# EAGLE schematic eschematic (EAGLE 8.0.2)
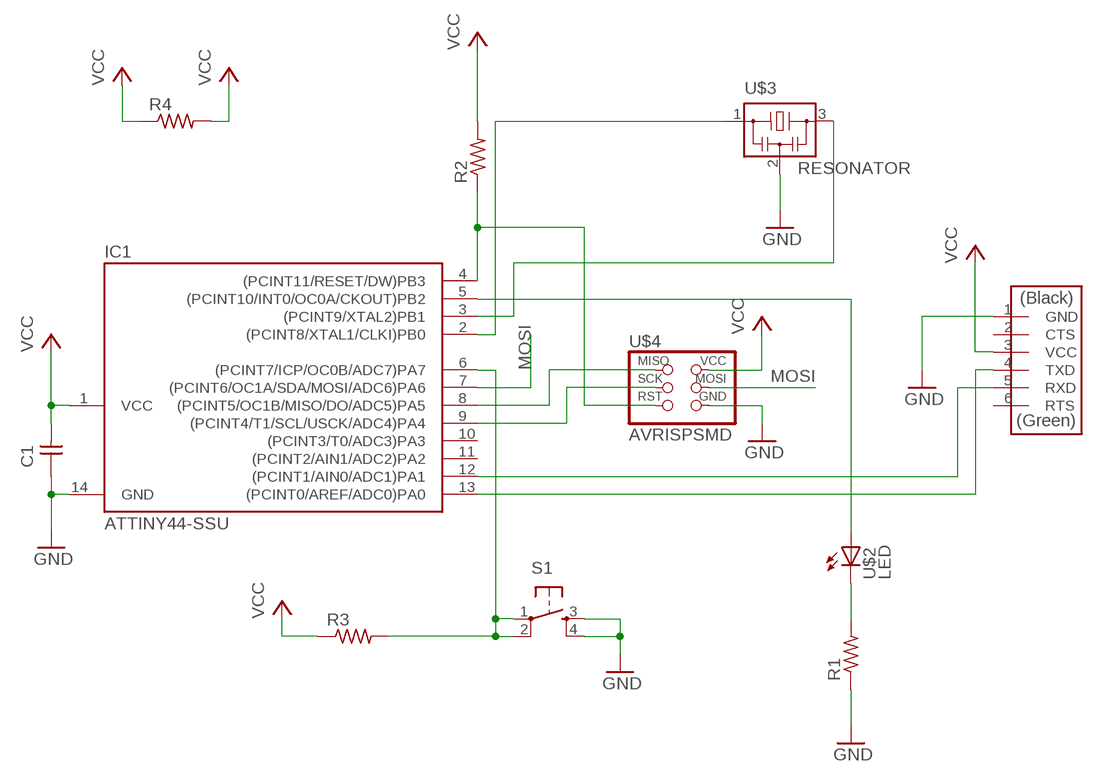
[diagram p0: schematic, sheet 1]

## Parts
C1  CAP-UNPOLARIZED  [C1206]
IC1  ATTINY44-SSU  [SOIC14]
R1  RES-US1206  [R1206]
R2  RES-US1206  [R1206]
R3  RES-US1206  [R1206]
R4  RES-US1206  [R1206]
S1  6MM_SWITCH6MM_SWITCH  [6MM_SWITCH]
U$1  FTDI-SMD-HEADER  [1X06SMD]
U$2  LED  [LED1206]
U$3  RESONATOR  [EFOBM]
U$4  AVRISPSMD  [2X03SMD]

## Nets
GND: C1.1 IC1.14(GND) R1.1 S1.3(S) S1.4(S1) U$1.1(GND) U$3.2 U$4.6(GND)
MOSI: IC1.7((PCINT6/OC1A/SDA/MOSI/ADC6)PA6) U$4.4(MOSI)
N$1: IC1.8((PCINT5/OC1B/MISO/DO/ADC5)PA5) U$4.1(MISO)
N$3: IC1.13((PCINT0/AREF/ADC0)PA0) U$1.4(TXD)
N$4: IC1.12((PCINT1/AIN0/ADC1)PA1) U$1.5(RXD)
N$5: IC1.9((PCINT4/T1/SCL/USCK/ADC4)PA4) U$4.3(SCK)
N$6: IC1.2((PCINT8/XTAL1/CLKI)PB0) U$3.1
N$7: IC1.3((PCINT9/XTAL2)PB1) U$3.3
N$8: IC1.5((PCINT10/INT0/OC0A/CKOUT)PB2) U$2.1(A)
N$9: R1.2 U$2.2(C)
N$10: IC1.6((PCINT7/ICP/OC0B/ADC7)PA7) R3.2 S1.1(P) S1.2(P1)
N$11: IC1.4((PCINT11/RESET/DW)PB3) R2.1 U$4.5(RST)
VCC: C1.2 IC1.1(VCC) R2.2 R3.1 R4.1 R4.2 U$1.3(VCC) U$4.2(VCC)
Unconnected: IC1.10((PCINT3/T0/ADC3)PA3) IC1.11((PCINT2/AIN1/ADC2)PA2) U$1.2(CTS) U$1.6(RTS)

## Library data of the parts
C1 = fab:CAP-UNPOLARIZED
IC1 = fab:ATTINY44
R1-R4 = fab:RES-US: Resistor (US Symbol)
S1 = fab:6MM_SWITCH: OMRON SWITCH
U$1 = fab:FTDI-SMD-HEADER
U$2 = fab:LED: LED
U$3 = fab:RESONATOR
U$4 = fab:AVRISP

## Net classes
0 default: width 0.35 mm, drill 0.4 mm, clearance 0.4 mm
